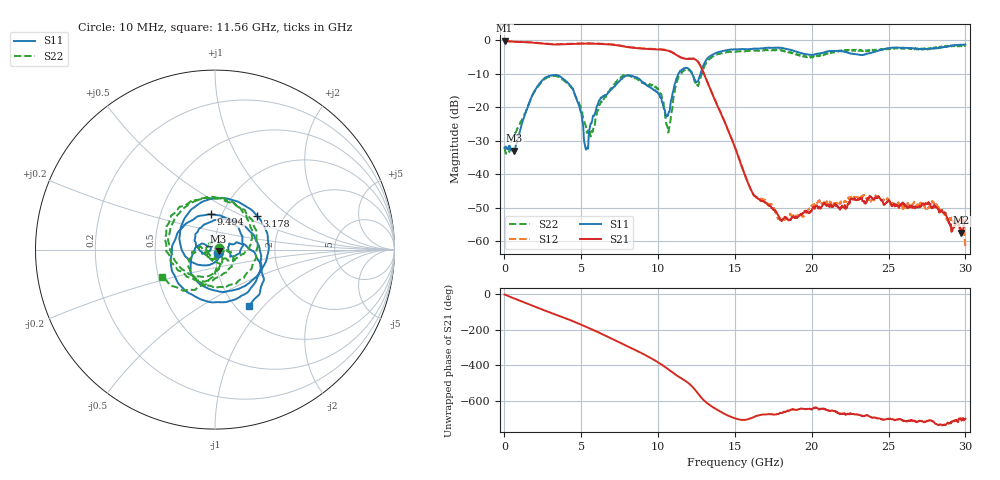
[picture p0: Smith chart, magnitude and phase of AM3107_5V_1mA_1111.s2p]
# Hz S DB R 50.0
!freq dBS11 angS11 dBS21 angS21 dBS12 angS12 dBS22 angS22
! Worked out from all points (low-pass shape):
!   1601 points, 10 MHz to 30 GHz, reference 50 ohm
!   highest |S21| = -0.12 dB at 10 MHz (marker M1); lowest = -57.5 dB at 29.74 GHz (marker M2)
!   |S21| within 3 dB of the highest: start of sweep to 10.64 GHz
!   lowest |S11| = -33.0 dB at 647.3 MHz (marker M3), VSWR 1.05, Z = 52 - j1.04 ohm
!   |S11| at or under -10 dB: start of sweep to 11.31 GHz; 12.21 GHz to 12.76 GHz (542.3 MHz wide, 4.34 % of centre)
!   |S22| runs from -34.0 to -1.5 dB; largest |S21 - S12| = 0.013
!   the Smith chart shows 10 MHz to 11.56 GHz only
!   S11 on the Smith chart (normalised r, x): 10 MHz: 1.04, -0.03; 3.178 GHz: 1.47, +0.60; 9.494 GHz: 0.89, +0.36; 11.56 GHz: 1.15, -0.83
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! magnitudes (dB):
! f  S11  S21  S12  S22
! 10 MHz  -32.1  -0.1  -0.1  -32.1
! 647.3 MHz  -33.0  -0.5  -0.4  -27.9
! 1.903 GHz  -15.5  -0.7  -0.6  -15.7
! 3.178 GHz  -10.5  -1.2  -1.2  -10.7
! 4.359 GHz  -14.0  -1.1  -1.0  -14.2
! 5.015 GHz  -22.1  -1.0  -0.9  -20.5
! 5.314 GHz  -32.7  -1.0  -0.9  -26.0
! 5.727 GHz  -23.4  -1.0  -0.9  -27.4
! 6.158 GHz  -18.0  -1.1  -1.0  -19.4
! 7.601 GHz  -11.7  -1.7  -1.6  -10.9
! 9.494 GHz  -14.1  -2.7  -2.5  -13.1
! 10.02 GHz  -16.1  -2.7  -2.6  -14.9
! 10.68 GHz  -21.7  -3.2  -3.1  -27.5
! 11.56 GHz  -8.7  -5.3  -5.2  -9.5
! 12.7 GHz  -10.9  -7.2  -7.1  -12.3
! 15.01 GHz  -2.7  -32.1  -31.9  -3.4
! 16.15 GHz  -2.6  -45.7  -45.7  -3.0
! 17.85 GHz  -2.3  -52.6  -53.0  -3.0
! 20.01 GHz  -4.4  -50.7  -49.5  -5.0
! 25.01 GHz  -2.4  -47.7  -48.0  -2.6
! 29.74 GHz  -1.4  -57.5  -53.1  -1.8
! 30 GHz  -1.2  -53.7  -61.5  -1.5
